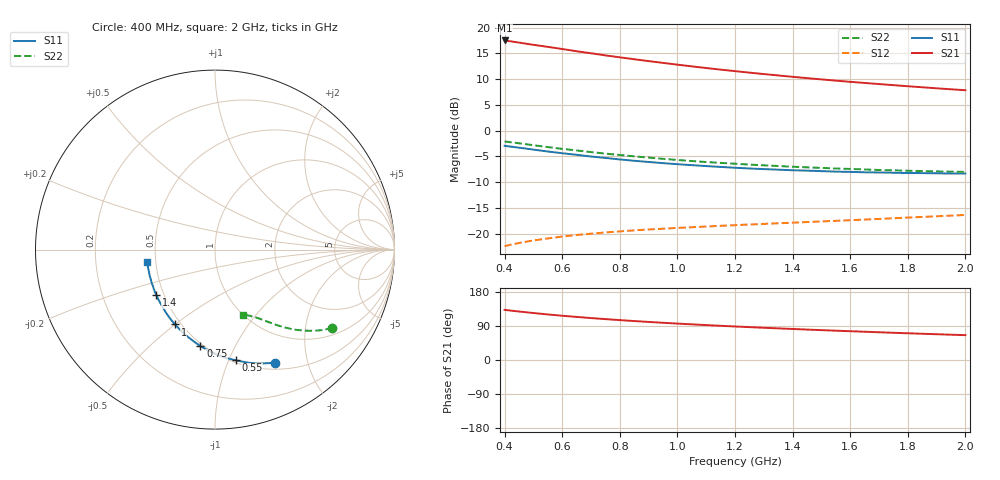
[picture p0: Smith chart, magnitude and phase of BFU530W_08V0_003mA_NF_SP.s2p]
! Filename:  P:\Prog\Test\Noise\ATS_data\Testdata_Net\06 Compressed Noise after Statistics\BFU530W_APM2013_09_A05_08p0V_003mA_NF_CM01_D.sf
! Date/Time: Tue 26/Mar/2013 18:06:04
! BFU530W_APM2013_09_A05_08p0V_1to25mA_NF_CM01_Bias3_R.sf
! Noise Parameter Data File
! BFU530W_APM2013_09_A05_08p0V_1to25mA_NF_CM01
! Date/time: Thu Mar 21 21:44:48 2013
! VAR V_out= 8.000000
! VAR I_out= 3.000000
! VAR V_in= 0.802800
! VAR I_in= 0.029905
! Device data file deembeded for feedlines and parallel
! Original file: \06 Compressed Noise after Statistics\BFU530W_APM2013_09_A05_08p0V_003mA_NF_CM01_R.sf
! Feed-files: PR019V01_070313_Feed1.s2p, PR019V01_070313_Feed2.s2p
! Parallel-file: PR019V01_070313_Par.s2p
# MHz S MA R 50
!  Freq-MHz  S11-mag  S11-arg  S21-mag  S21-arg  S12-mag  S12-arg  S22-mag  S22-arg
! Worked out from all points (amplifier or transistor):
!   37 points, 400 MHz to 2 GHz, reference 50 ohm
!   highest |S21| = 17.5 dB at 400 MHz (marker M1)
!   |S21| within 3 dB of that: start of sweep to 763.6 MHz
!   unconditionally stable (mu >= 1): nowhere
!   at 500 MHz: K = 0.36, MSG = 19.0 dB, |S12| = -21.3 dB
!   at 1.1 GHz: K = 0.70, MSG = 15.4 dB, |S12| = -18.6 dB
!   at 2 GHz: K = 0.99, MSG = 12.1 dB, |S12| = -16.4 dB
!   lowest NFmin = 0.52 dB at 420 MHz
!   S11 on the Smith chart (normalised r, x): 400 MHz: 0.59, -1.50; 550 MHz: 0.52, -1.06; 750 MHz: 0.48, -0.74; 1 GHz: 0.47, -0.50; 1.4 GHz: 0.45, -0.28; 2 GHz: 0.45, -0.07
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400  0.7137 -61.9  7.515 132.3  0.07564 58.2  0.7859 -33.6
420  0.701 -64.5  7.378 130.4  0.07797 57.2  0.7729 -34.8
440  0.6894 -66.9  7.237 128.8  0.08016 56.3  0.7601 -35.8
480  0.6668 -71.6  6.946 125.6  0.08409 54.6  0.7352 -37.8
500  0.6549 -74.0  6.821 124.0  0.08589 53.8  0.7225 -38.6
550  0.6277 -79.4  6.513 120.2  0.08994 52.2  0.693 -40.8
600  0.6045 -84.7  6.21 116.8  0.09374 50.7  0.6661 -42.6
650  0.5829 -89.4  5.904 113.7  0.09713 49.5  0.6429 -44.2
700  0.5613 -94.3  5.645 110.6  0.1 48.5  0.6198 -45.8
750  0.5438 -98.6  5.383 107.9  0.1027 47.7  0.599 -47.0
800  0.5257 -102.9  5.154 105.3  0.1053 47.0  0.5809 -48.3
850  0.5102 -107.0  4.938 102.8  0.1076 46.5  0.563 -49.4
950  0.4843 -114.5  4.551 98.2  0.1117 45.7  0.533 -51.4
1000  0.4727 -118.1  4.375 96.1  0.1137 45.5  0.5195 -52.2
1100  0.4532 -124.8  4.058 92.2  0.1173 45.4  0.4963 -54.0
1200  0.4367 -131.0  3.786 88.5  0.1209 45.4  0.4775 -55.5
1300  0.4236 -136.9  3.546 85.1  0.1244 45.6  0.4607 -56.9
1400  0.4129 -142.4  3.335 81.9  0.1279 46.0  0.4466 -58.3
1500  0.4048 -147.6  3.147 78.8  0.1315 46.5  0.4353 -59.8
1600  0.3982 -152.5  2.981 76.0  0.1352 47.2  0.4253 -61.1
1750  0.3905 -159.3  2.767 71.9  0.1412 48.3  0.4126 -63.1
2000  0.3841 -169.8  2.47 65.5  0.152 50.1  0.3978 -66.7
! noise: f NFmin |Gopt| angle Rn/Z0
400  0.5251  0.3718  26.88  0.1424
460  0.5432  0.3552  32.23  0.1398
600  0.5682  0.3536  39.21  0.1456
800  0.6249  0.337  54.72  0.1288
1000  0.6775  0.3548  64.76  0.1274
1200  0.7293  0.3383  78.58  0.1196
1400  0.7279  0.3192  90.02  0.1169
1600  0.7326  0.3266  109.9  0.089
1800  0.811  0.3308  120.3  0.0872
2000  0.8971  0.327  133.5  0.0779
